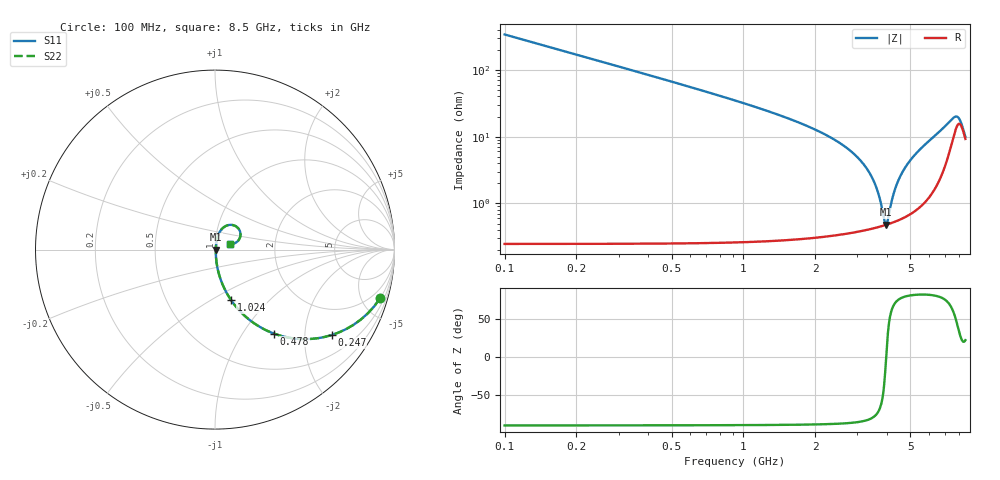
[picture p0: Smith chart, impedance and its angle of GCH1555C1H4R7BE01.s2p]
!Murata Part Number: GCH1555C1H4R7BE01
!These Parameters are Measured in Series Mode Connection
!Data Generated on Jun 19, 2026
!  o--ll--o
!Port1  Port2
!  o------o
!Operation Temp=25[degC], DC Bias Voltage=0[V]
!Freq. Start=100[MHz] Stop=9[GHz] 401[Steps]
# Hz S RI R 50
!Freq.(Hz) S11(Real) S11(Imag) S21(Real) S21(Imag) S12(Real) S12(Imag) S22(Real) S22(Imag)
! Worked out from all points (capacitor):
!   401 points, 100 MHz to 8.5 GHz, reference 50 ohm
!   read as one part in series: C = 4.7 pF near 142 MHz
!   lowest |Z| = 480 mohm at 3.964 GHz (marker M1)
!   series resonance near 3.96 GHz, so ESL is about 340 pH
!   S11 on the Smith chart (normalised r, x): 100 MHz: 1.00, -6.77; 247 MHz: 1.00, -2.73; 478 MHz: 1.01, -1.40; 1.024 GHz: 1.01, -0.62; 8.5 GHz: 1.18, +0.08
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1e8  0.9195 -0.2717  0.0805 0.2717  0.0805 0.2717  0.9195 -0.2717
2.47e8  0.6507 -0.4758  0.3493 0.4758  0.3493 0.4758  0.6507 -0.4758
4.78e8  0.3284 -0.4678  0.6716 0.4678  0.6716 0.4678  0.3284 -0.4678
7.09e8  0.1777 -0.3795  0.8223 0.3795  0.8223 0.3795  0.1777 -0.3795
1.024e9  0.0892 -0.2809  0.9108 0.2809  0.9108 0.2809  0.0892 -0.2809
1.507e9  0.0384 -0.1851  0.9616 0.1851  0.9616 0.1851  0.0384 -0.1851
2.914e9  0.00658 -0.0538  0.9934 0.0538  0.9934 0.0538  0.00658 -0.0538
3.271e9  0.00511 -0.0335  0.9949 0.0335  0.9949 0.0335  0.00511 -0.0335
3.523e9  0.00466 -0.0205  0.9953 0.0205  0.9953 0.0205  0.00466 -0.0205
3.712e9  0.00458 -0.0114  0.9954 0.0114  0.9954 0.0114  0.00458 -0.0114
3.901e9  0.00469 -0.00265  0.9953 0.00265  0.9953 0.00265  0.00469 -0.00265
3.964e9  0.00477 0.000181  0.9952 -0.000181  0.9952 -0.000181  0.00477 0.000181
4.006e9  0.00483 0.00205  0.9952 -0.00205  0.9952 -0.00205  0.00483 0.00205
4.3e9  0.0055 0.0147  0.9945 -0.0147  0.9945 -0.0147  0.0055 0.0147
4.531e9  0.0063 0.0243  0.9937 -0.0243  0.9937 -0.0243  0.0063 0.0243
4.825e9  0.00769 0.0362  0.9923 -0.0362  0.9923 -0.0362  0.00769 0.0362
5.707e9  0.0151 0.0713  0.9849 -0.0713  0.9849 -0.0713  0.0151 0.0713
7.114e9  0.0607 0.1319  0.9393 -0.1319  0.9393 -0.1319  0.0607 0.1319
7.576e9  0.1096 0.1333  0.8904 -0.1333  0.8904 -0.1333  0.1096 0.1333
7.87e9  0.1399 0.0992  0.8601 -0.0992  0.8601 -0.0992  0.1399 0.0992
8.122e9  0.1337 0.0557  0.8663 -0.0557  0.8663 -0.0557  0.1337 0.0557
8.5e9  0.0856 0.0315  0.9144 -0.0315  0.9144 -0.0315  0.0856 0.0315
